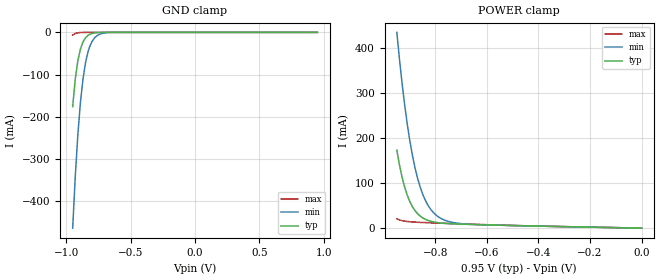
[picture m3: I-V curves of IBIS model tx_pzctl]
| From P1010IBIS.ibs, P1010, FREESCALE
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[Model] tx_pzctl
Model_type Input
Vinh=0.76
Vinl=0.19
C_comp   1.67pF   1.67pF   1.67pf
[Model Spec]
[Temperature Range] 65   125   -40
[Voltage Range]   0.95   0.85   1.21
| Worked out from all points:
|   GND clamp passes 1 mA (typ) near -0.77 V on its own axis
|   POWER clamp passes 1 mA (typ) near -0.09 V on its own axis
[GND Clamp]
-950mV    -175.9mA   -463.9mA   -6.552mA
-930mV    -111.2mA   -341.7mA   -2.735mA
-910mV    -67.53mA   -242.8mA   -1.068mA
-890mV    -39.71mA   -166.4mA   -361.8uA
-870mV    -22.75mA   -110.4mA   -66.85uA
-850mV    -12.73mA   -71.2mA    0A
-820mV    -5.084mA   -35.33mA   0A
-800mV    -2.652mA   -21.61mA   0A
-760mV    -602.9uA   -7.614mA   0A
-720mV    -25.41uA   -2.369mA   0A
-640mV    0A         0A         0A
950mV     0A         0A         0A
[POWER Clamp]
-950mV    173.1mA    434.7mA    20.55mA
-930mV    113.8mA    323.3mA    16.69mA
-920mV    91.7mA     275.5mA    15.58mA
-900mV    59.46mA    195.6mA    14.19mA
-880mV    39.27mA    135.4mA    13.37mA
-860mV    27.04mA    92.24mA    12.79mA
-840mV    19.77mA    62.57mA    12.31mA
-820mV    15.48mA    42.86mA    11.87mA
-800mV    12.93mA    30.08mA    11.45mA
-750mV    10.04mA    14.91mA    10.44mA
-680mV    8.431mA    9.084mA    9.086mA
0V        706.6nA    753.3nA    331.3nA
